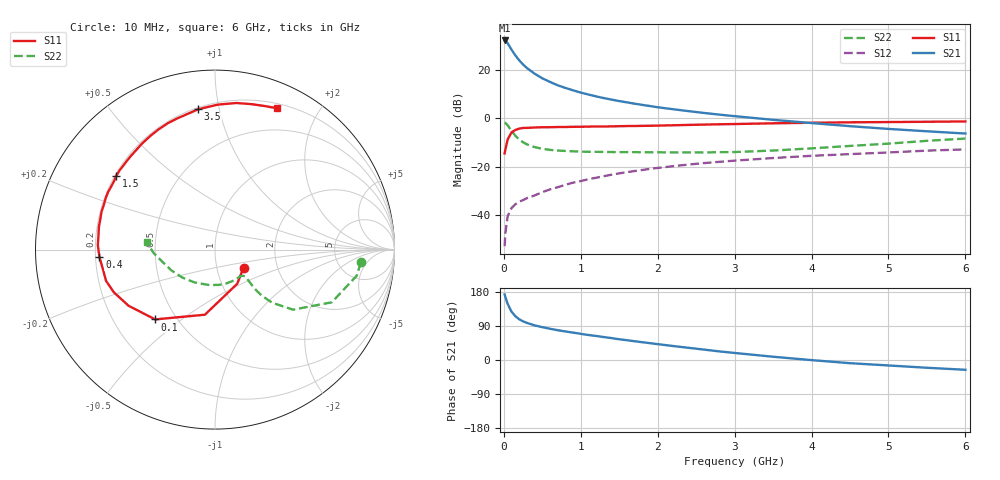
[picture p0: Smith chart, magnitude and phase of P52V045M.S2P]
! SIEMENS Small Signal Semiconductors
! BFP183
! Si NPN RF Bipolar Junction Transistor in SOT143
! VCE = 2 V  IC = 45 mA
! Common Emitter S-Parameters:  March  1996
# GHz  S  MA  R  50
!  f  S11  S21  S12  S22
! GHz  MAG  ANG  MAG  ANG  MAG  ANG  MAG  ANG
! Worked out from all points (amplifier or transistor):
!   36 points, 10 MHz to 6 GHz, reference 50 ohm
!   highest |S21| = 32.1 dB at 10 MHz (marker M1)
!   |S21| within 3 dB of that: start of sweep to 84.84 MHz
!   unconditionally stable (mu >= 1): start of sweep to 19.48 MHz; 271.5 MHz to end of sweep
!   at 250 MHz: K = 0.95, MSG = 28.0 dB, |S12| = -33.8 dB
!   at 1.4 GHz: K = 1.51, MAG = 11.3 dB, |S12| = -23.3 dB
!   at 6 GHz: K = 1.17, MAG = 0.8 dB, |S12| = -12.8 dB
!   S11 on the Smith chart (normalised r, x): 10 MHz: 1.35, -0.28; 100 MHz: 0.38, -0.40; 400 MHz: 0.22, -0.03; 1.5 GHz: 0.21, +0.32; 3.5 GHz: 0.21, +0.87; 6 GHz: 0.25, +1.51
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0.01  0.1882 -32.2  40.27 173.0  0.0023 78.0  0.8164 -5.0
0.02  0.2272 -57.0  39.72 166.4  0.0043 68.3  0.8023 -10.5
0.05  0.3671 -98.8  35.18 148.0  0.0096 66.3  0.7138 -24.3
0.1  0.5122 -130.6  26.02 127.5  0.0141 51.7  0.5483 -37.6
0.15  0.5744 -147.0  19.76 115.4  0.0169 48.6  0.4354 -42.9
0.2  0.6117 -157.1  15.68 107.5  0.0191 47.9  0.3649 -44.6
0.25  0.6316 -164.0  12.85 102.0  0.0205 48.7  0.3202 -44.6
0.3  0.6331 -169.1  10.88 97.9  0.0225 50.4  0.2894 -44.0
0.4  0.6453 -176.3  8.31 91.4  0.0256 53.3  0.2541 -42.8
0.5  0.6533 177.8  6.667 86.6  0.0299 55.5  0.2348 -42.2
0.6  0.6543 172.8  5.615 82.4  0.0341 57.5  0.2233 -42.1
0.7  0.6593 168.8  4.79 78.6  0.0378 59.1  0.2157 -42.7
0.9  0.6664 161.6  3.773 72.3  0.047 59.8  0.2082 -44.9
1.1  0.6731 154.8  3.088 66.0  0.0555 60.2  0.2035 -48.2
1.5  0.6863 143.1  2.263 54.7  0.0731 58.6  0.2004 -56.9
1.8  0.697 134.7  1.888 46.9  0.0858 56.5  0.1989 -65.1
2.2  0.7169 124.6  1.537 36.9  0.1028 52.9  0.1971 -77.0
2.8  0.7517 110.4  1.19 22.7  0.1264 46.7  0.1999 -97.2
3.5  0.7875 96.8  0.929 8.6  0.1513 39.9  0.2159 -122.4
4.5  0.8254 81.7  0.687 -8.4  0.1822 29.7  0.2688 -154.4
5.5  0.8465 70.9  0.539 -20.5  0.215 20.7  0.3424 -176.8
6  0.8602 66.2  0.484 -25.8  0.2281 15.6  0.3819 174.0
